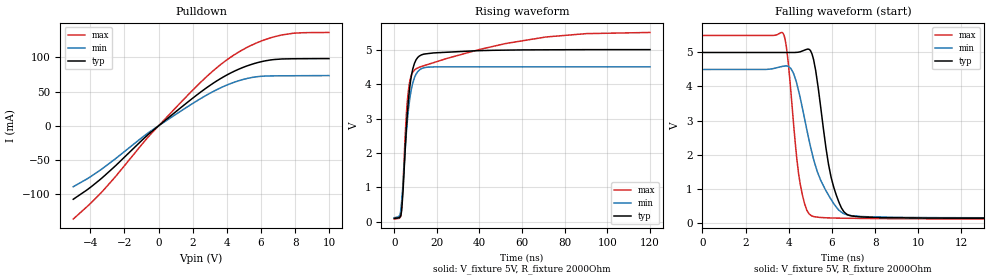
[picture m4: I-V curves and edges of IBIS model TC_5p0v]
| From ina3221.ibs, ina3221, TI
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|   TC_5p0v model
[Model]   TC_5p0v
Model_type   Open_drain
Polarity   Non-Inverting
Vmeas = 2.5
Vref = 5
Cref = 1pF
Rref = 2000
|   typ   min   max
C_comp   0.609pF   0.575pF   0.639pF
[Voltage Range]   5   4.5   5.5
[Temperature Range]   30   88   -40
[Pullup Reference]   5   4.5   5.5
[Pulldown Reference]   -0   -0   -0
[Power Clamp Reference]   5   4.5   5.5
[GND Clamp Reference]   -0   -0   -0
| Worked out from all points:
|   slope of the pulldown table from 0 to 0.75 V, typ, clamps not added: 48.9 ohm
|   falling waveform, V_fixture 5V, R_fixture 2000Ohm: 20-80 % time 710ps typ, 1.12ns min, 501ps max; typ from 5 V to 0.119 V
|   rising waveform, V_fixture 5V, R_fixture 2000Ohm: 20-80 % time 3.22ns typ, 3.42ns min, 5.47ns max; typ from 0.101 V to 5 V
[Pulldown]
|   Voltage   I(typ)   I(min)   I(max)
-5V       -107.1mA   -88.82mA   -135.9mA
-4.16V    -92.82mA   -76.89mA   -117.1mA
-3.245V   -74.49mA   -61.49mA   -94.34mA
-575mV    -11.88mA   -9.653mA   -15.34mA
1.48V     30.09mA    24.38mA    38.75mA
2.83V     55.84mA    45.06mA    72.13mA
3.97V     73.76mA    59.17mA    95.67mA
4.705V    82.72mA    65.86mA    107.8mA
5.455V    89.73mA    70.48mA    117.7mA
6.76V     96.72mA    72.91mA    129.8mA
7.915V    97.88mA    73.1mA     135.1mA
9.985V    98.15mA    73.35mA    136.2mA
[Ramp]
R_load = 2000
|   typ   min   max
dV/dt_r   2.93899/3.21973e-09   2.62728/3.41561e-09   3.24936/5.45022e-09
dV/dt_f   2.92858/7.1002e-10   2.62135/1.1215e-09   3.23849/5.00808e-10
[Falling Waveform]
V_fixture = 5V
V_fixture_min = 4.5V
V_fixture_max = 5.5V
R_fixture = 2000Ohm
C_fixture = 0F
|   Time   V(typ)   V(min)   V(max)
0s        5V         4.5V       5.5V
3.745ns   5V         4.595V     5.557V
3.974ns   5V         4.596V     4.712V
4.532ns   5.021V     3.662V     1.122V
5.079ns   4.955V     2.042V     192.1mV
5.433ns   3.619V     1.317V     151mV
5.843ns   1.706V     805mV      137mV
6.32ns    603.9mV    363.7mV    129.1mV
7.464ns   161mV      175.4mV    120.6mV
120ns     119mV      131.1mV    102.5mV
[Rising Waveform]
V_fixture = 5V
V_fixture_min = 4.5V
V_fixture_max = 5.5V
R_fixture = 2000Ohm
C_fixture = 0F
|   Time   V(typ)   V(min)   V(max)
0s        101.3mV    121.1mV    82.37mV
2.598ns   137.7mV    191.6mV    121.3mV
3.28ns    254mV      467.7mV    257.7mV
4.157ns   933.2mV    1.131V     1.136V
5.591ns   2.609V     2.495V     3.025V
6.98ns    3.736V     3.421V     3.972V
8.748ns   4.45V      4.04V      4.347V
11.77ns   4.814V     4.406V     4.489V
71.19ns   4.995V     4.5V       5.367V
120ns     5V         4.5V       5.498V
